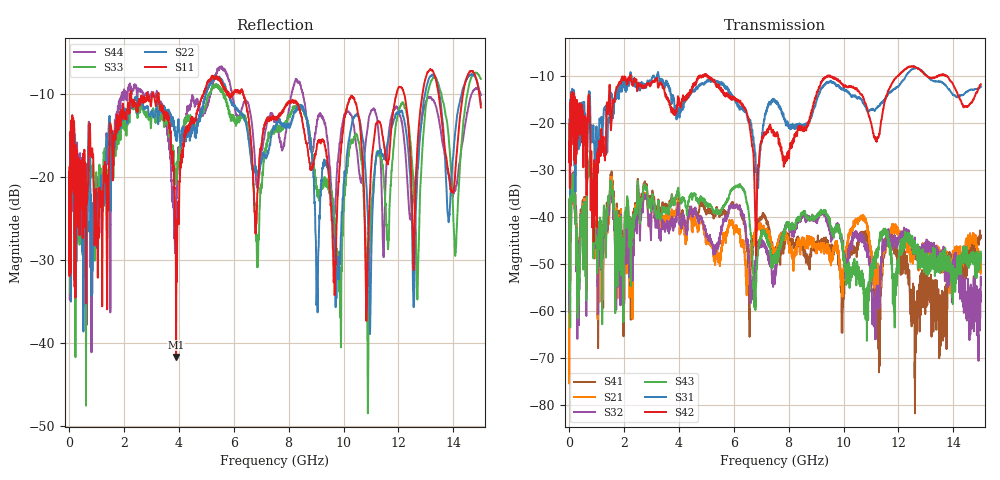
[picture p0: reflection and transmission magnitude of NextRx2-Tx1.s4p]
! FILE: N:\QM 2007\Prüfprotokolle\Highspeed\Konfektionierte Ltg\L45593-D106\D30\8216\0002\Next\NextRx2-Tx1.s4p
# MHz S DB R 50.00
! FREQ  S11  S12  S13  S14
!  S21  S22  S23  S24
!  S31  S32  S33  S34
!  S41  S42  S43  S44
!  DB  ANG  DB  ANG  DB  ANG  DB  ANG
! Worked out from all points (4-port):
!   2999 points, 10 MHz to 15 GHz, reference 50 ohm
!   strongest paths, dB at 10 MHz, 3.755 GHz, 7.505 GHz, 11.26 GHz, 15 GHz:
!     S42: -24.1, -16.7, -22.4, -23.0, -11.7
!     S31: -23.8, -14.2, -15.2, -16.3, -12.2
!     S43: -42.8, -35.2, -49.3, -47.9, -47.3
!     S32: -46.8, -39.9, -51.9, -57.1, -54.4
!     S21: -44.7, -38.7, -49.3, -51.0, -52.0
!     S41: -54.0, -35.1, -46.6, -62.0, -43.9
!   lowest |S11| = -41.7 dB at 3.905 GHz (marker M1), VSWR 1.02, Z = 50.8 + j0.312 ohm
!   |S11| at or under -10 dB: start of sweep to 2.245 GHz; 3.268 GHz to 4.914 GHz (1.647 GHz wide, 40.3 % of centre); 6.337 GHz to 11.94 GHz (5.599 GHz wide, 61.3 % of centre)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
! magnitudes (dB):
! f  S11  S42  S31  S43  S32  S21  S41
! 10 MHz  -19.4  -24.1  -23.8  -42.8  -46.8  -44.7  -54.0
! 3.905 GHz  -41.7  -17.1  -17.6  -35.5  -40.2  -38.6  -35.4
! 6.81 GHz  -25.7  -46.7  -30.0  -53.7  -48.2  -42.8  -42.1
! 10.46 GHz  -11.2  -12.4  -14.5  -52.7  -43.6  -40.4  -46.4
! 10.88 GHz  -29.5  -17.2  -17.5  -57.7  -46.3  -43.3  -44.9
! 12.61 GHz  -22.8  -8.0  -8.3  -46.3  -46.5  -48.1  -67.4
! 15 GHz  -11.7  -11.7  -12.2  -47.3  -54.4  -52.0  -43.9
